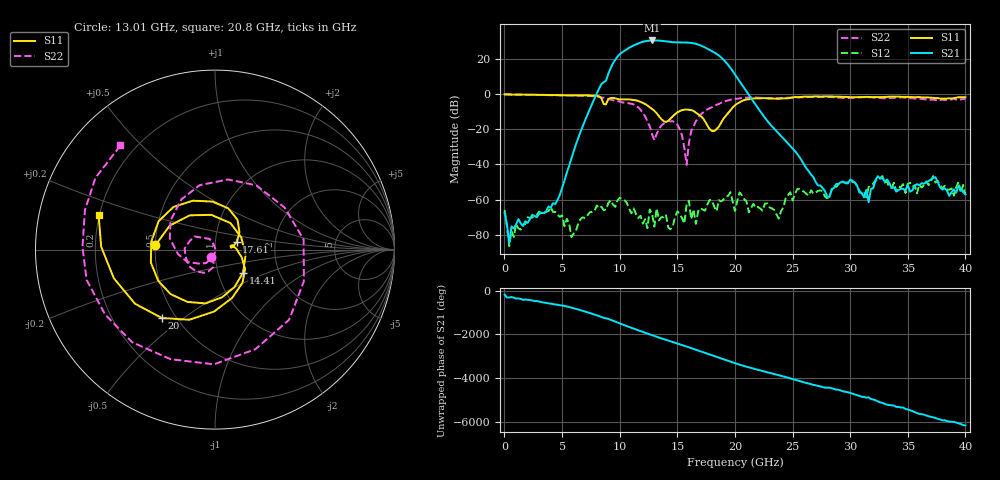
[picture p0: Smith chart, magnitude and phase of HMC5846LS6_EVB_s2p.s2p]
! Analog Devices, Inc.
! 20 Alpha Road
! Chelmsford, MA 01824
! http://www.analog.com
! Tel: 978-250-3343
! Fax: 978-250-3373
! Device:	HMC5846LS6
! Description:	GaAs pHEMT MMIC 2 WATT POWER AMPLIFIER WITH POWER DETECTOR, 12 - 16 GHz
! Conditions:	Vdd = Vdd1 = Vdd2 = Vdd3 = Vdd4 = Vdd5 = Vdd6 = 7 V
!		Vgg = Vgg1 = -0.708 V
!		Idd = 1204 mA
!		Pin = -10 dBm
!		Tamb = +25 C
! Product validation SN 5, measured on evaluation board EVAL01-HMC5846L56 (PCB 128996-2)
! Measurements referenced to the evaluation board coaxial connectors
# GHz S DB R 50
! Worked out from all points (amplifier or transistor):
!   201 points, 10 MHz to 40 GHz, reference 50 ohm
!   highest |S21| = 30.5 dB at 12.81 GHz (marker M1)
!   |S21| within 3 dB of that: 11.15 GHz to 17.07 GHz (5.92 GHz wide, 41.9 % of centre)
!   unconditionally stable (mu >= 1): start of sweep to end of sweep
!   at 6.608 GHz: K = 493.60, MAG = -5.1 dB, |S12| = -70.9 dB
!   at 20 GHz: K = 103.22, MAG = 15.7 dB, |S12| = -66.5 dB
!   at 40 GHz: K = 42773.65, MAG = -49.1 dB, |S12| = -57.4 dB
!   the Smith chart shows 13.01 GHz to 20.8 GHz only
!   S11 on the Smith chart (normalised r, x): 13.01 GHz: 0.50, +0.03; 14.41 GHz: 1.32, -0.35; 17.61 GHz: 1.27, +0.11; 20 GHz: 0.42, -0.42; 20.8 GHz: 0.20, +0.14
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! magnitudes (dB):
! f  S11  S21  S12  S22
! 10 MHz  -0.1  -67.6  -65.9  -0.1
! 409.9 MHz  -0.2  -84.9  -86.5  -0.2
! 4.409 GHz  -0.6  -62.5  -67.0  -0.7
! 5.809 GHz  -0.7  -36.5  -81.3  -0.7
! 6.808 GHz  -0.7  -17.9  -70.1  -0.8
! 9.808 GHz  -2.7  21.4  -60.4  -3.9
! 12.81 GHz  -8.4  30.5  -68.1  -22.9
! 13.01 GHz  -9.5  30.5  -75.4  -26.2
! 13.41 GHz  -12.5  30.4  -71.8  -20.0
! 14.41 GHz  -13.9  29.7  -76.9  -15.5
! 15.81 GHz  -8.8  29.3  -62.8  -40.3
! 16.21 GHz  -9.1  29.1  -71.1  -21.0
! 17.61 GHz  -17.9  25.9  -62.7  -8.7
! 20 GHz  -6.3  11.1  -66.5  -2.7
! 20.2 GHz  -5.4  9.2  -60.6  -2.6
! 20.8 GHz  -3.4  3.4  -59.8  -2.1
! 23.8 GHz  -2.6  -22.5  -70.9  -2.3
! 24.8 GHz  -2.1  -29.5  -55.8  -2.1
! 26.8 GHz  -1.4  -47.2  -56.7  -1.5
! 31.6 GHz  -1.6  -61.5  -52.8  -1.8
! 33.4 GHz  -1.5  -50.6  -53.1  -2.2
! 40 GHz  -1.8  -57.0  -57.4  -2.9
